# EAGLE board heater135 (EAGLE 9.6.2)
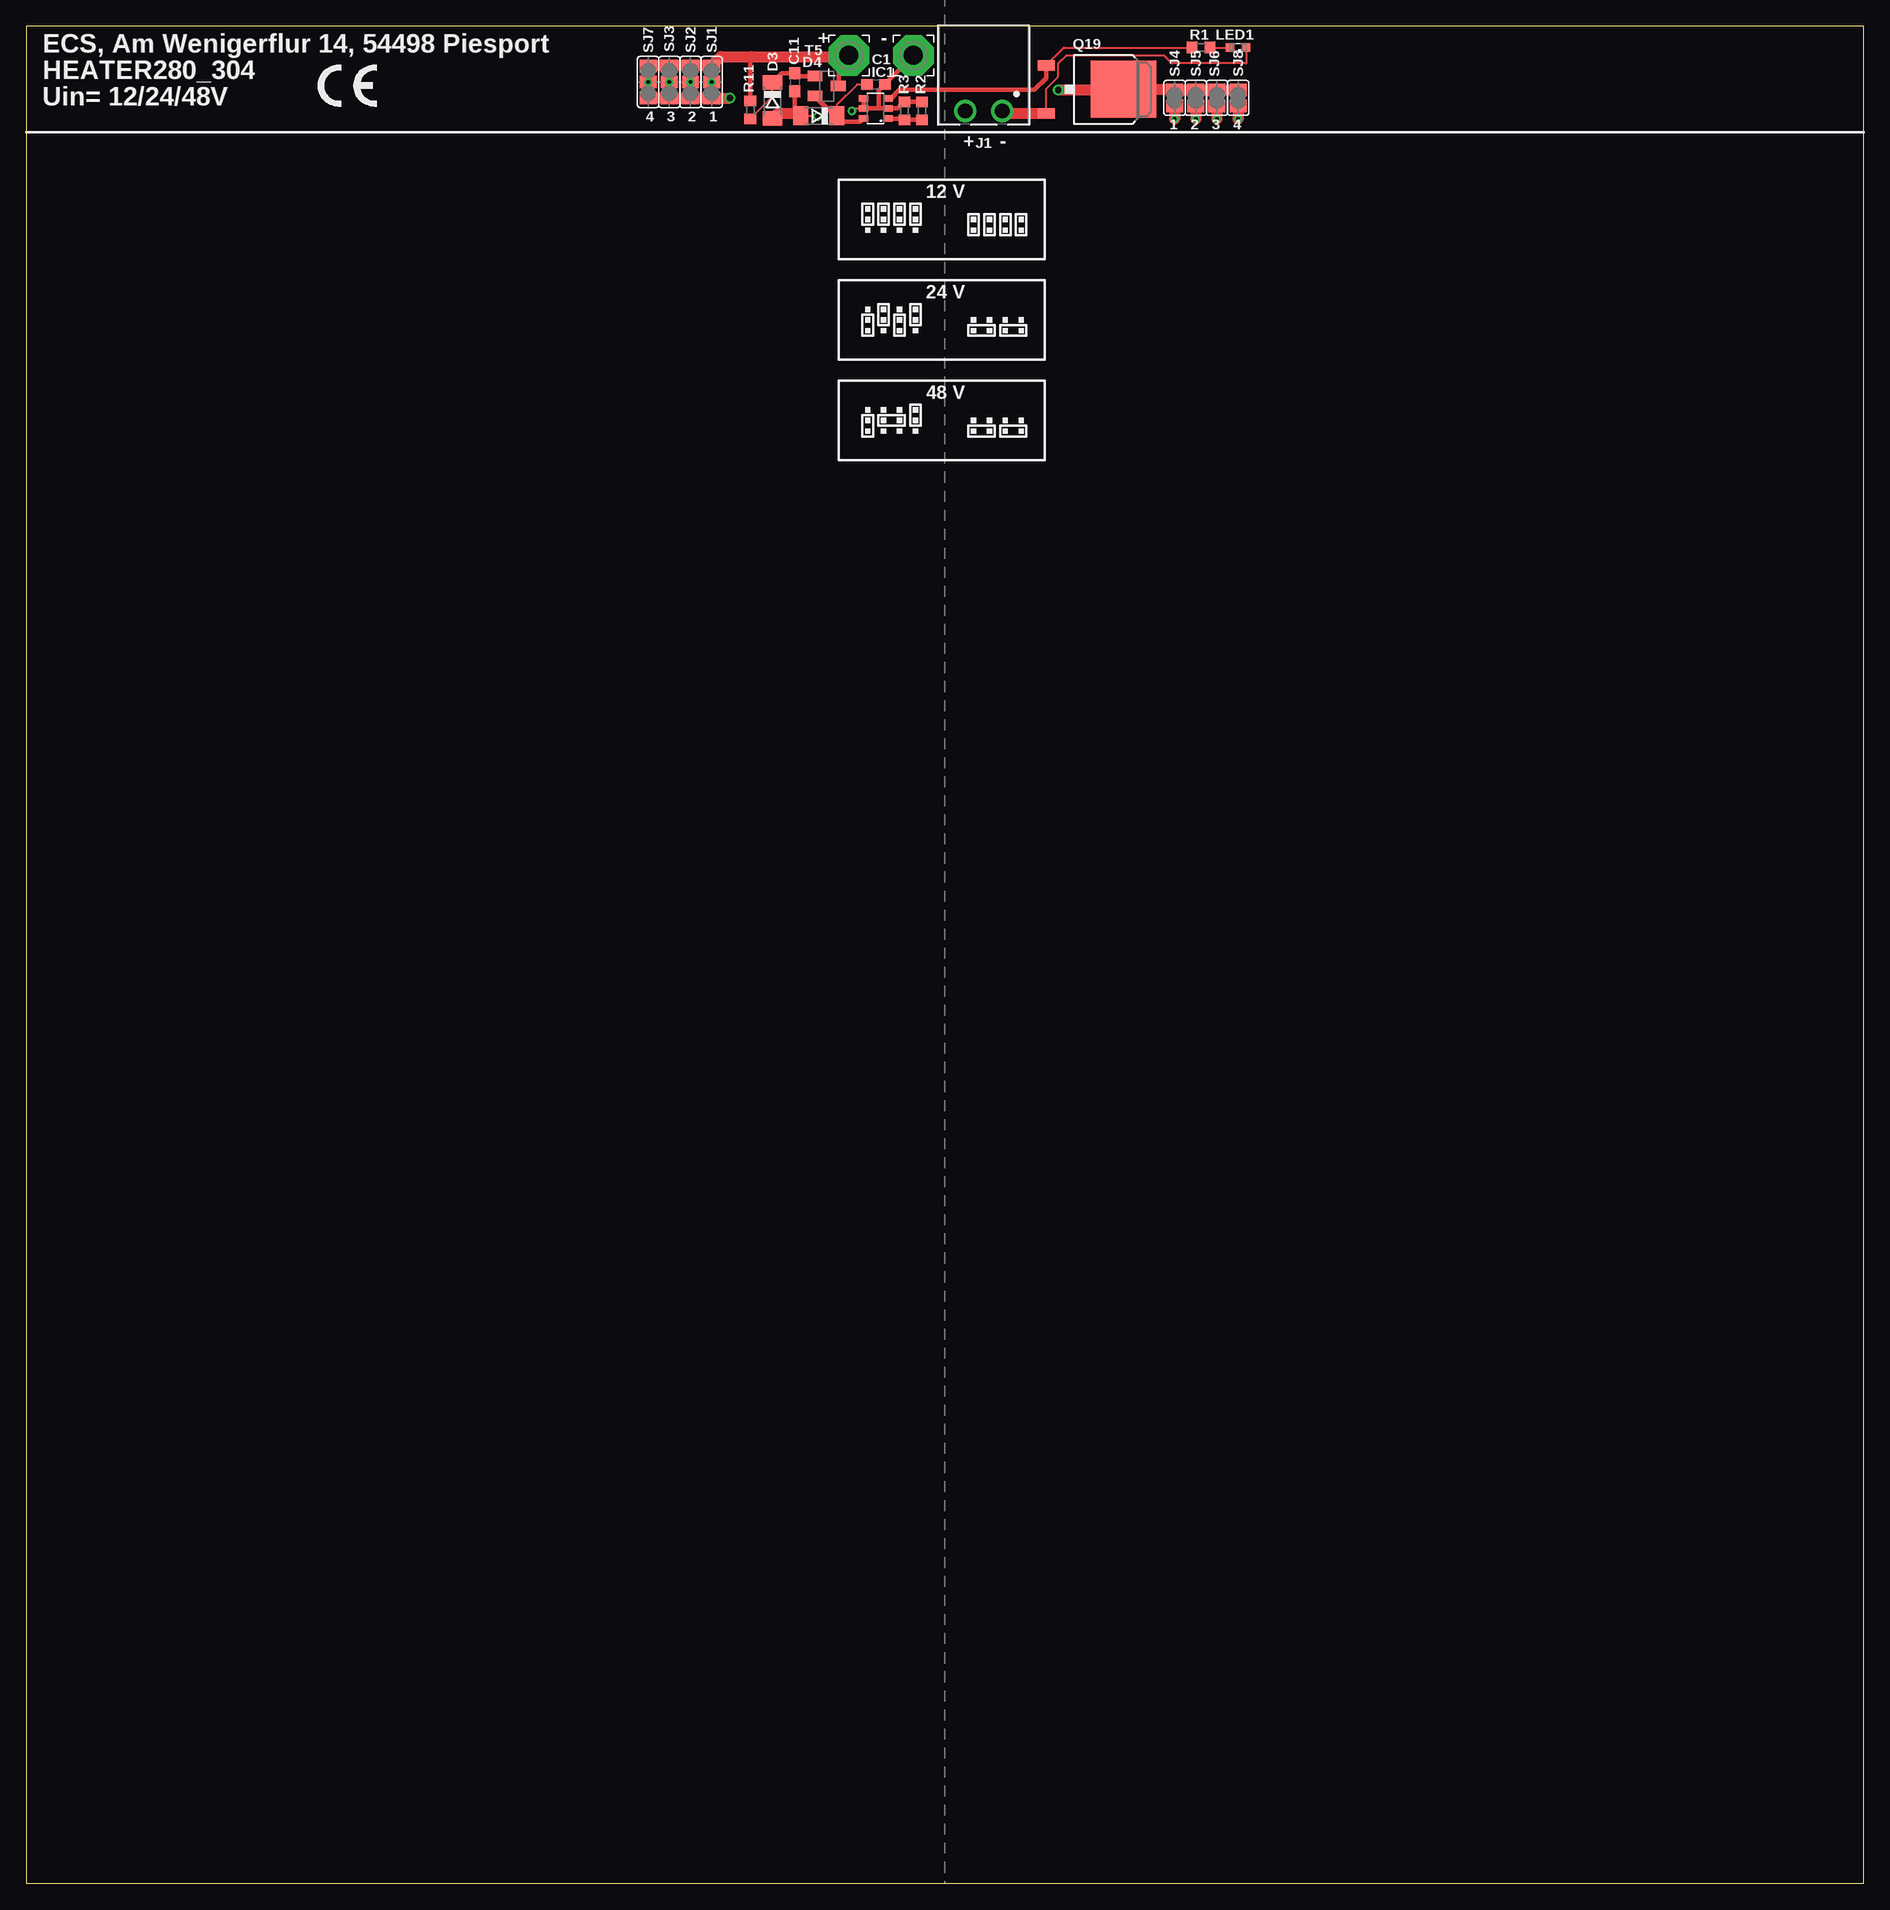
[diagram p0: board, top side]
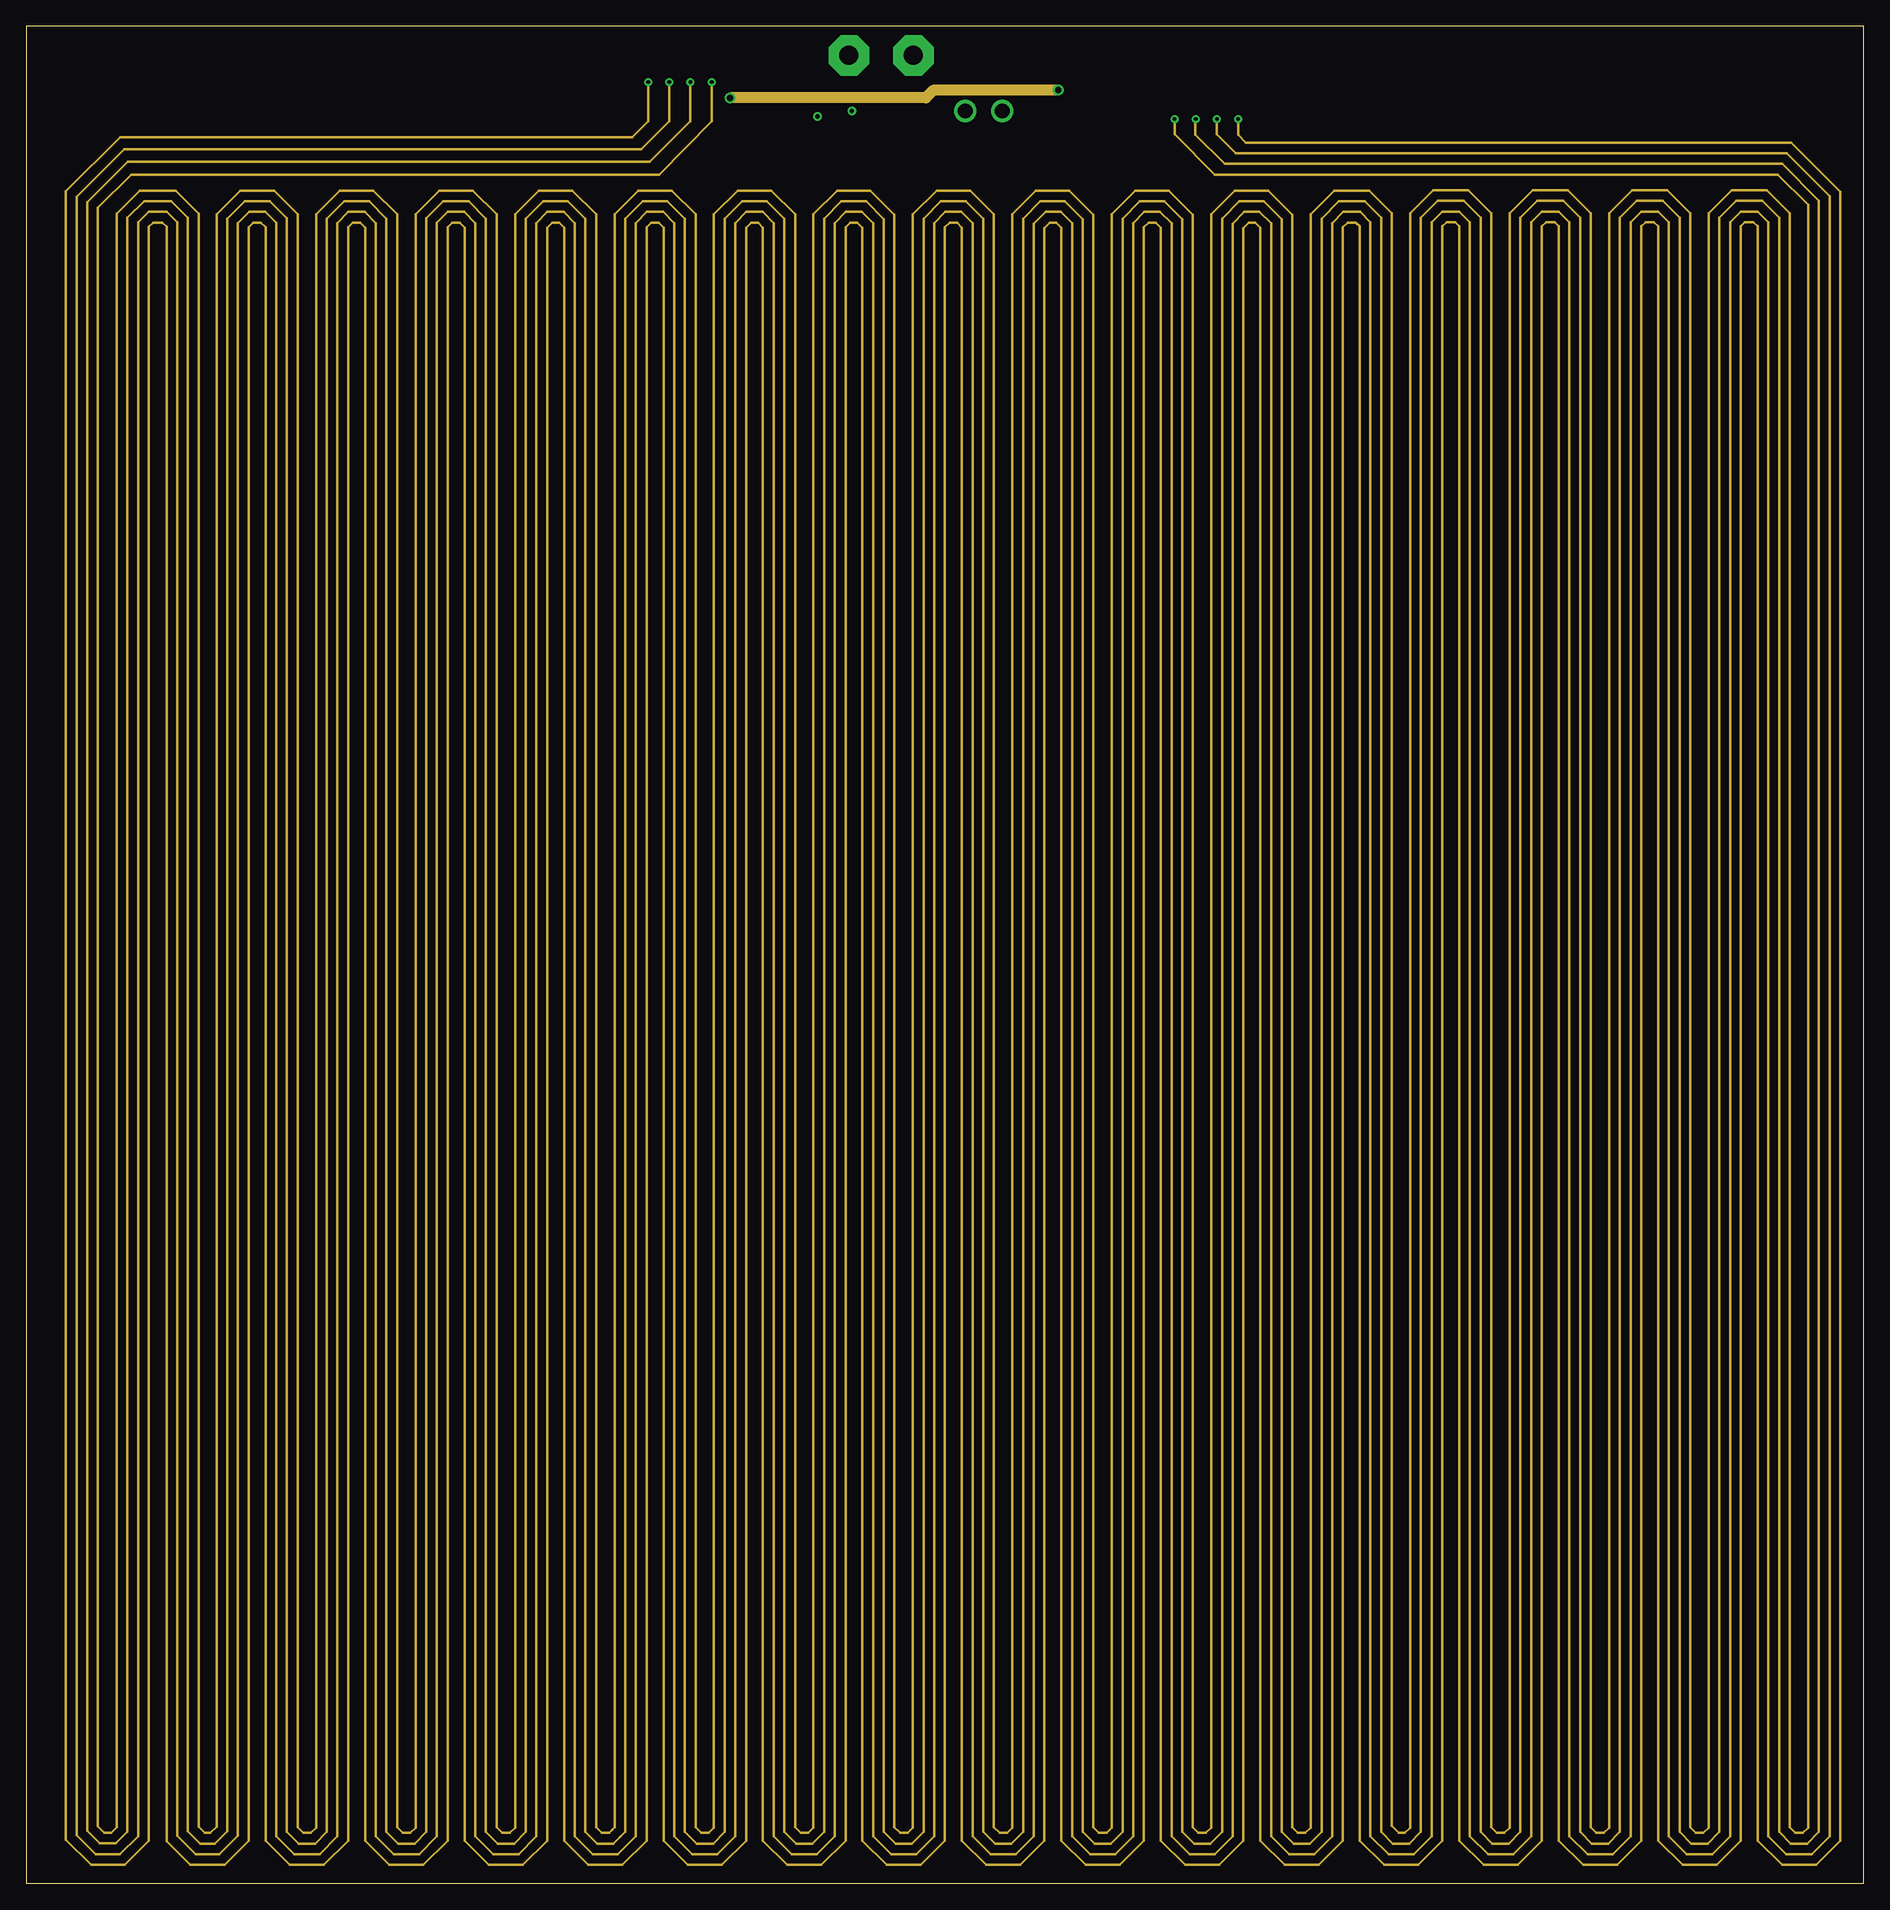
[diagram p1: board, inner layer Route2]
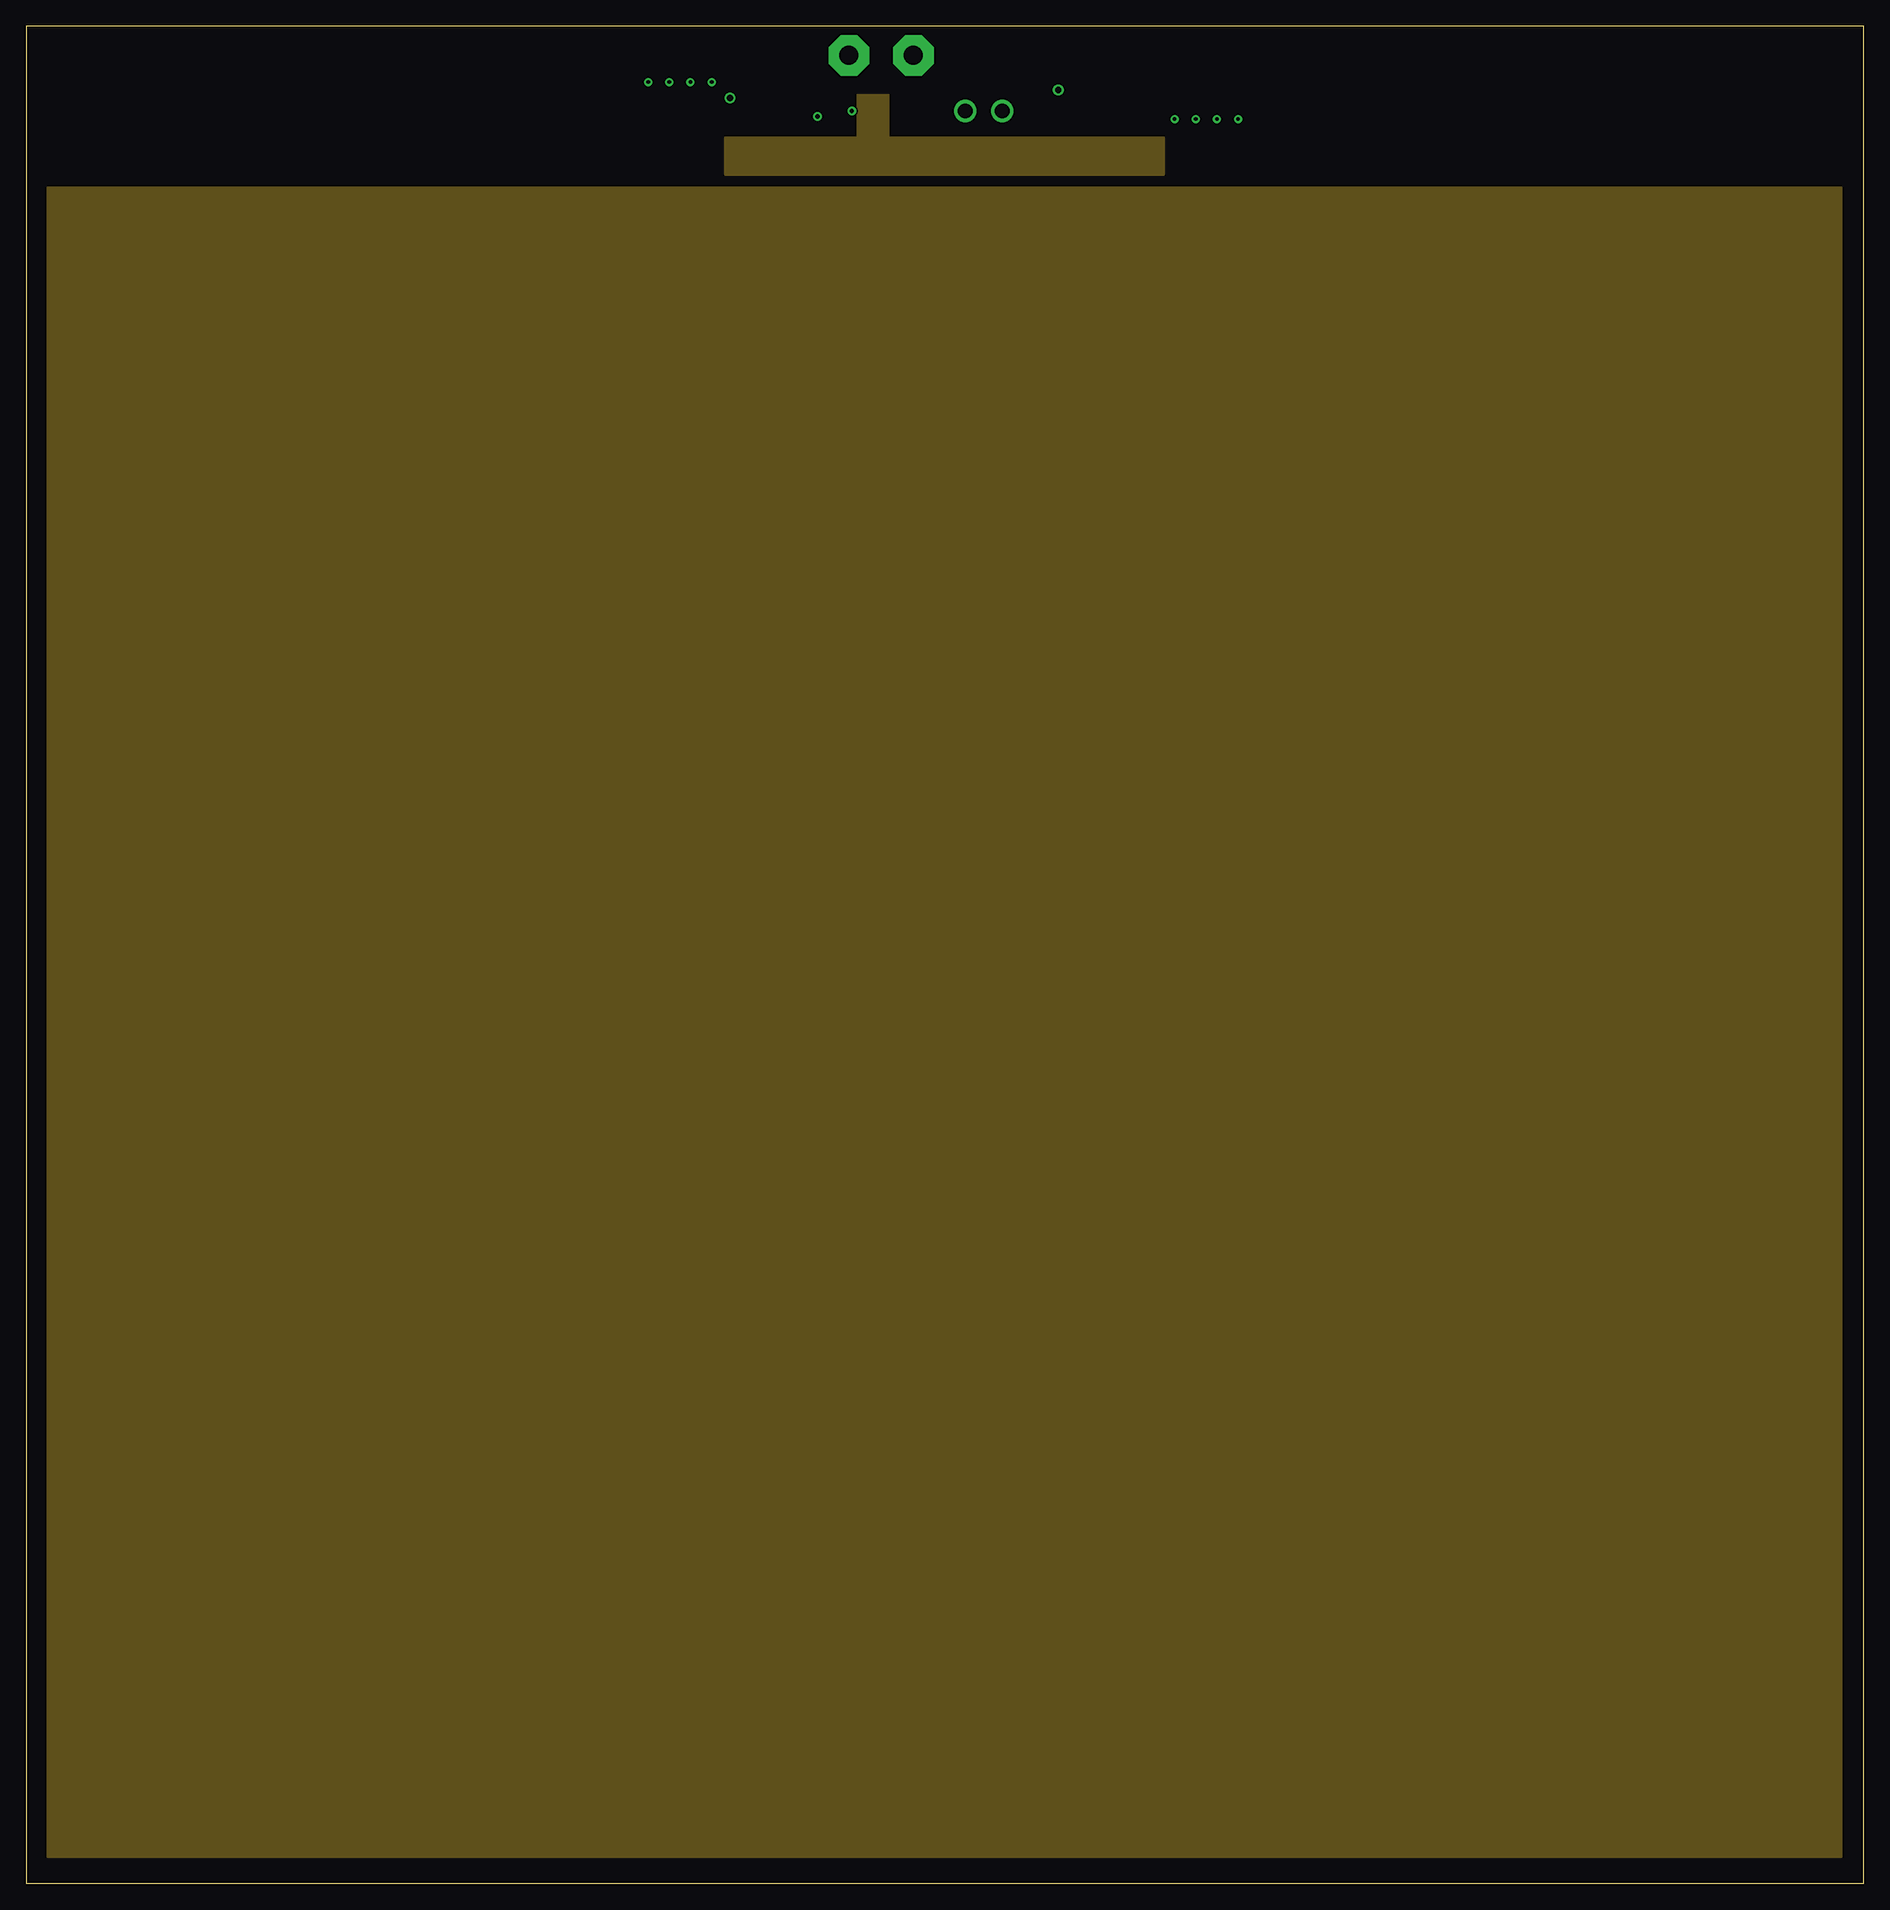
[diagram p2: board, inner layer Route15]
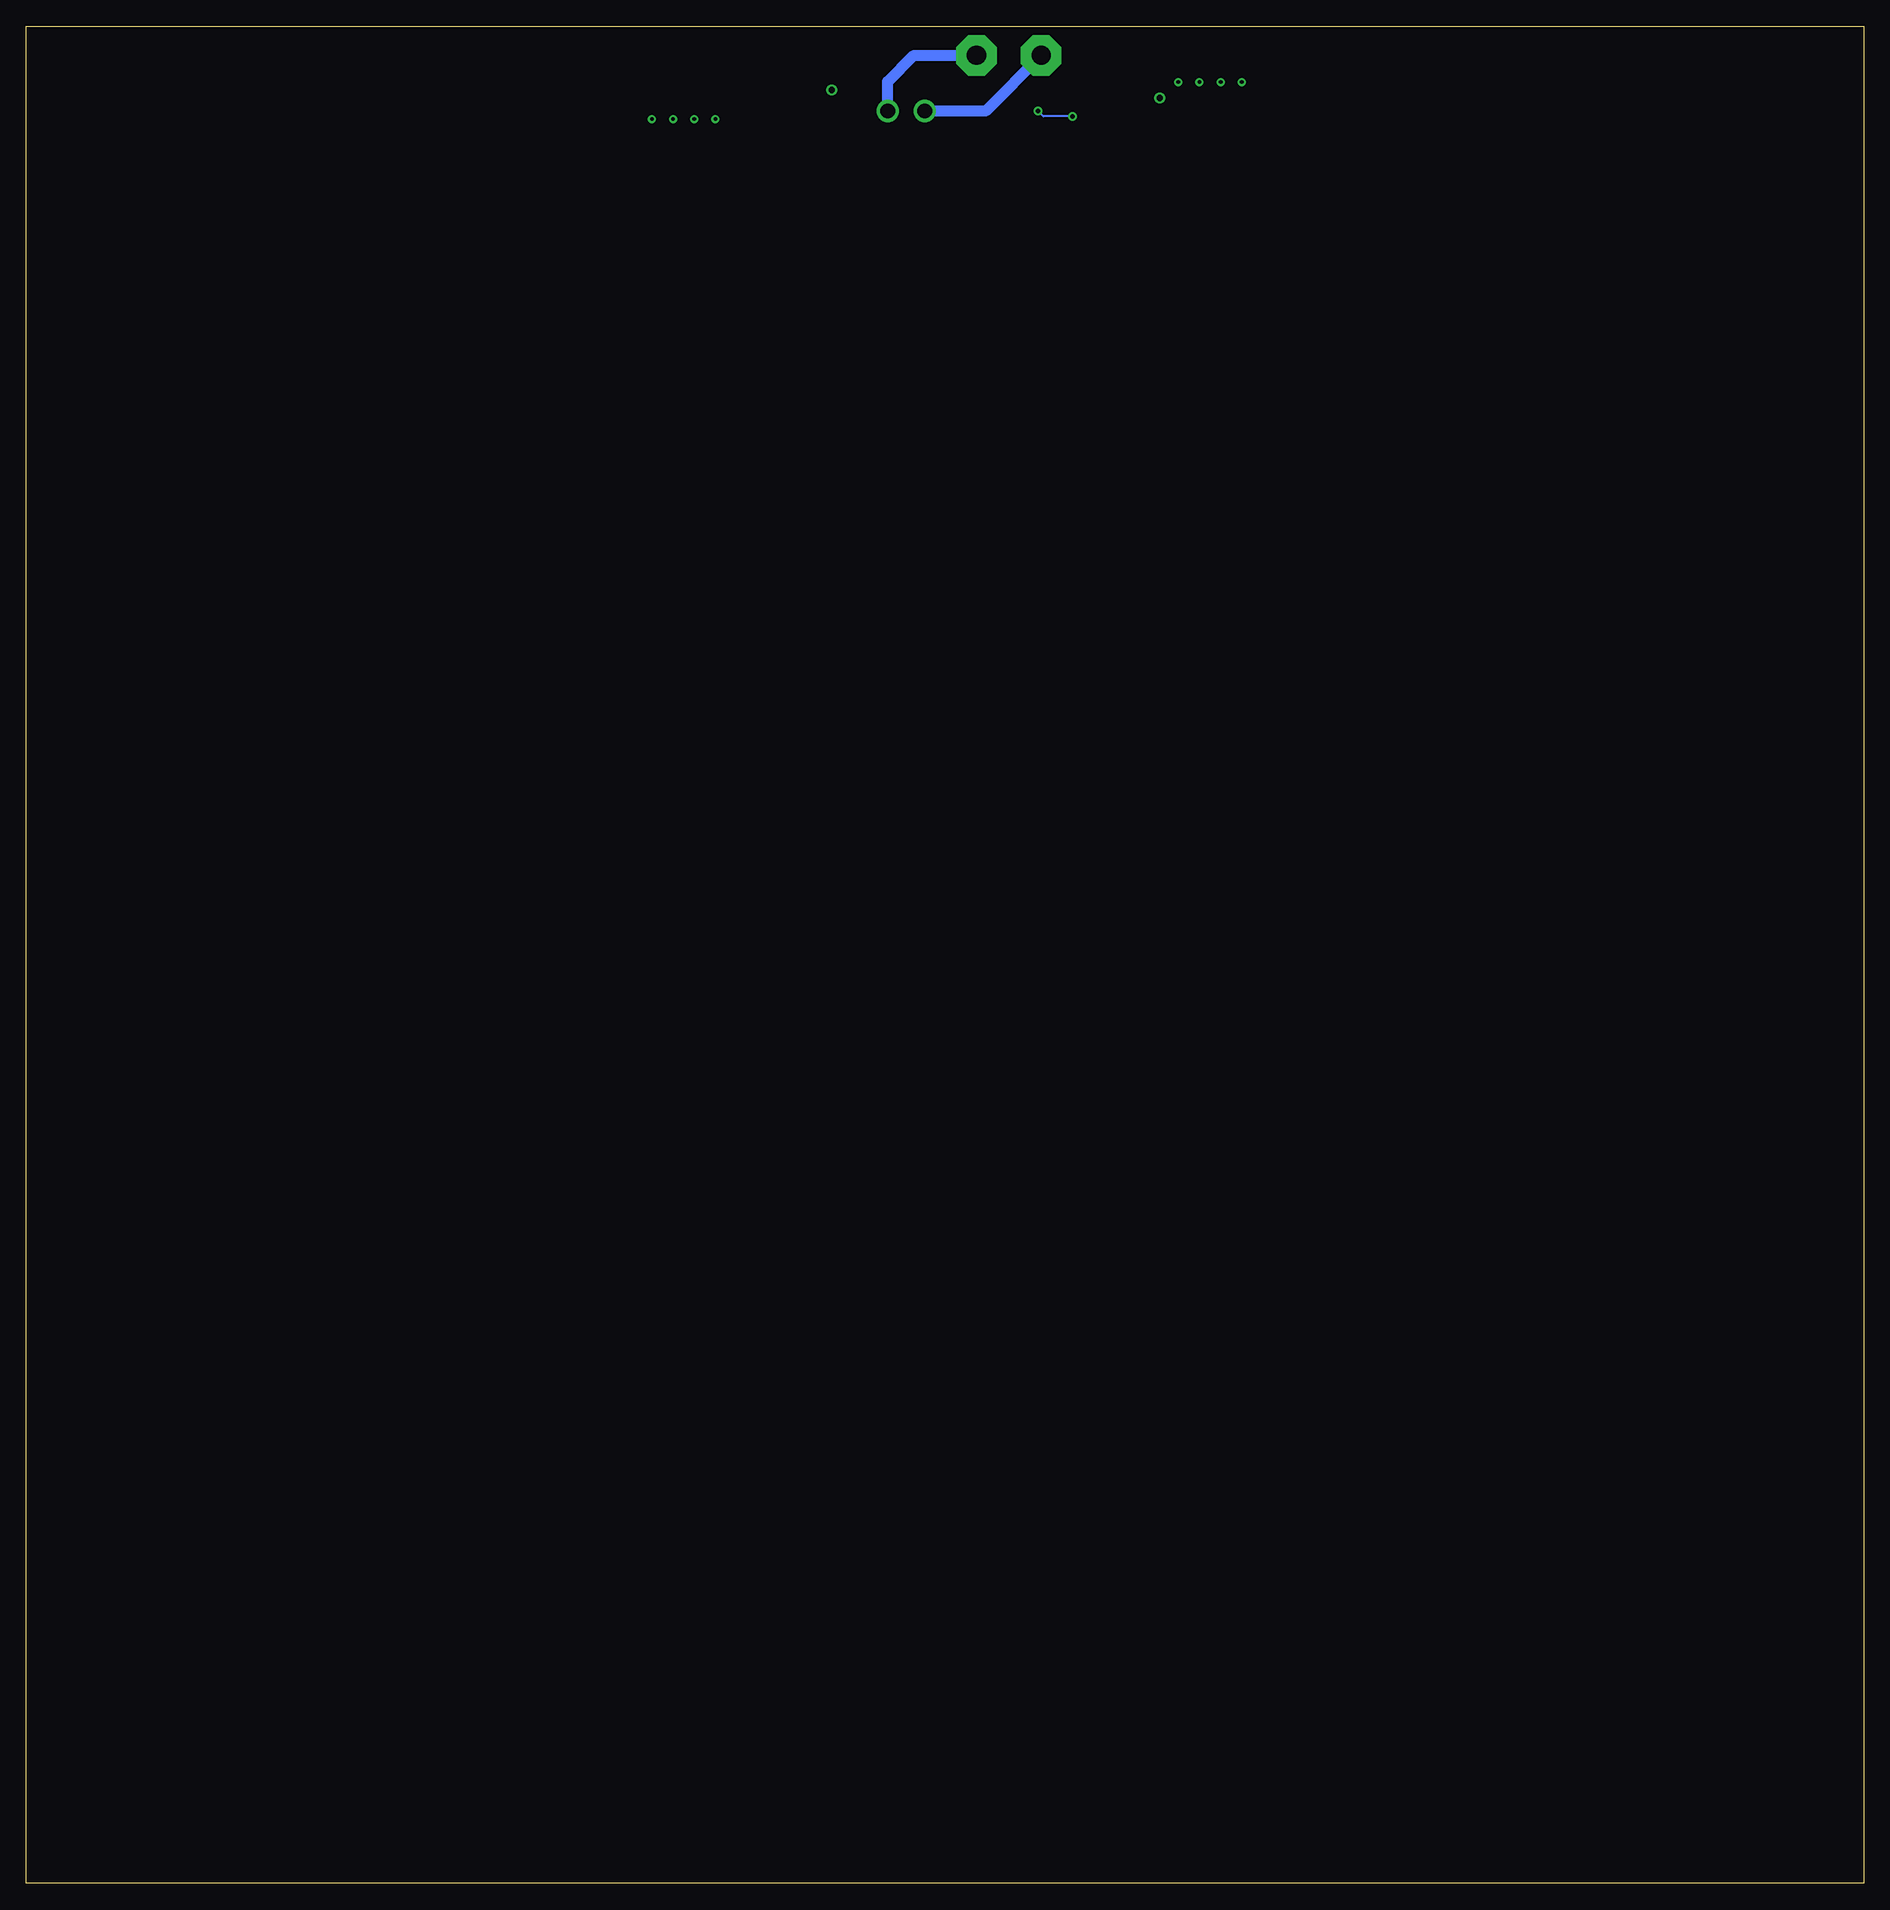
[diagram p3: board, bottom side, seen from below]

Size 173.6 x 175.5 mm. Coordinates in mm from the lower left corner, seen from the top.
Outline: 0,0 173.6,0 173.6,175.5 0,175.5 0,0
Copper layers (1+2*15+16): Top 0.035mm / dielectric 1.5mm / Route2 0.0175mm / dielectric 0.15mm / Route15 0.0175mm / dielectric 0.2mm / Bottom 0.035mm
Design rules "default *": minimum track width 6mil, minimum drill 0.35mm, track to track 6mil, track to pad 6mil, pad to pad 6mil, via to via 6mil, smd to smd 6mil, copper to edge 40mil, drill to drill 6mil, minimum pad ring 10mil, minimum via ring 8mil, stop-mask expansion 4mil, vias tented up to drill 0mil, thermal gap 10mil

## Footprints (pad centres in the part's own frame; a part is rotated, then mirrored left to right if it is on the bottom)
C0603 = smd 1.1 x 1: 1 -0.85,0; 2 0.85,0
SOD80C = smd 1.4 x 1.8: A 1.7,0; C -1.7,0
SOT23-6 = smd 0.6 x 0.9: 1 -0.95,-1.15; 2 0,-1.15; 3 0.95,-1.15; 4 0.95,1.15; 5 0,1.15; 6 -0.95,1.15
691322110002 = drill 1.4: 1 -1.75,0; 2 1.75,0
SML0603 = smd 0.8 x 0.8: A 0.75,0; C -0.75,0
3,81/1,4 = drill 1.8 pad 3.81 octagon: 1 0,0
D-PACK = smd 1 x 1.6: 1 -2.28,-4.8; 3 2.28,-4.8 | smd 5.4 x 6.2: 4 0,2.5
R0603 = smd 1 x 1.1: 1 -0.85,0; 2 0.85,0
SJ_2 = smd 1.168 x 1.6: 1 -1.524,0; 2 0,0; 3 1.524,0
SJ = smd 1.168 x 1.6: 1 -0.762,0; 2 0.762,0
SOT23-BEC = smd 1 x 1.4: B -0.95,-1.1; C 0,1.1; E 0.95,-1.1

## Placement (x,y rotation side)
C1  100n  [C0603]  80.27,170.02 0 top
C11  100n  [C0603]  72.6,170.23 270 top
D3  5V6  [SOD80C]  70.5,168.5 270 top
D4  5V1  [SOD80C]  74.88,167.05 180 top
IC1  MCP9510H  [SOT23-6]  80.25,167.75 90 top
J1  [691322110002]  90.46,167.51 180 top
LED1  [SML0603]  114.5,173.5 180 top
PAD1  [3,81/1,4]  77.72,172.76 0 top
PAD2  [3,81/1,4]  83.82,172.76 0 top
Q19  IRLR3110Z  [D-PACK]  101.16,169.55 270 top
R1  10k  [R0603]  111,173.5 180 top
R2  82k  [R0603]  84.64,167.52 270 top
R3  2M2  [R0603]  82.97,167.52 270 top
R11  100k  [R0603]  68.4,167.62 90 top
SJ1  [SJ_2]  64.75,170.25 90 top
SJ2  [SJ_2]  62.75,170.25 90 top
SJ3  [SJ_2]  60.75,170.25 90 top
SJ4  [SJ]  108.5,168.75 270 top
SJ5  [SJ]  110.5,168.75 270 top
SJ6  [SJ]  112.5,168.75 270 top
SJ7  [SJ_2]  58.75,170.25 90 top
SJ8  [SJ]  114.5,168.75 270 top
T5  BSR19A  [SOT23-BEC]  75.61,169.86 270 top
U$1  [CE-4MM]  27.5,167.88 0 top

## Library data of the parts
C1 C11 = rcl; PARTNO: C067; SPICEPREFIX: C
D3 = diode; PARTNO: D013
D4 = diode; PARTNO: D012
IC1 = mcp9509; PARTNO: IC333
J1 = Wurth_Connectors_WR-TBL Pluggable Connector; DATASHEET-URL: https://www.we-online.com/catalog/datasheet/691322110002.pdf; IR-UL: 10A; IR-VDE: 10.5A; MOUNT: THT; PART-NUMBER: 691322110002; PARTNO: CON212; PINS: 2; PITCH: 3.5mm; TYPE: Horizontal; WORKING-VOLTAGE-UL: 300V (AC); WORKING-VOLTAGE-VDE: 300V (AC)
LED1 = led; PARTNO: D078
PAD1 PAD2 = wirepad
Q19 = IRFR2607; PARTNO: T086
R1 = rcl; PARTNO: R221; SPICEPREFIX: R
R2 = rcl; PARTNO: R243; SPICEPREFIX: R
R3 = rcl; PARTNO: R277; SPICEPREFIX: R
R11 = rcl; PARTNO: R245; SPICEPREFIX: R
SJ1-SJ8 = jumper
T5 = transistor-neu-to92; PARTNO: T056
U$1 = logo

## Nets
+UB: J1.2 PAD1.1 R11.2 SJ1.3 SJ2.3 SJ3.3 SJ7.3 T5.C
GND: C1.2 C11.2 D3.A D4.A IC1.2 IC1.4 IC1.5 J1.1 LED1.C PAD2.1 Q19.3 R2.1 R3.1
N$1: IC1.3 Q19.1 R1.2
N$2: SJ1.2 SJ4.2
N$3: C11.1 D3.C R11.1 T5.B
N$4: IC1.1 R2.2 R3.2
N$5: C1.1 D4.C IC1.6 T5.E
N$6: LED1.A R1.1
N$7: SJ2.2 SJ5.2
N$8: SJ3.2 SJ6.2
N$9: SJ7.2 SJ8.2
N$11: Q19.4 SJ1.1 SJ2.1 SJ3.1 SJ4.1 SJ5.1 SJ6.1 SJ7.1 SJ8.1

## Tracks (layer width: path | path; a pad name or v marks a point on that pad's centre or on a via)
+UB
  Top 0.406: T5.C 76.75,169.9 76.75,171.79 77.61,172.65 PAD1.1 | R11.2 68.4,172.54 68.5,172.65
  Top 1.016: SJ7.3 SJ3.3 SJ2.3 SJ1.3 65.62,172.65 68.5,172.65 77.61,172.65
  Bottom 1.016: PAD1.1 82.97,167.51 J1.2
GND  (via drill 0.4)
  Top 0.2: LED1.C 115.25,172 108.25,172 107.5,172.75 98.25,172.75 97.5,172 97.5,170.75 96.36,169.61 Q19.3 | D4.A 74.7,167.05 v74.75,167 | v78,167.5 78.25,167.75 IC1.5
  Top 0.406: D4.A 72.6,167.63 C11.2 | 80.56,167.75 IC1.2 82.35,167.75 R3.1 R2.1 | 80.56,167.75 80.56,169.46 C1.2 81.12,170.06 PAD2.1 | IC1.4 IC1.5 80.56,167.75
  Top 1.016: D3.A 70.95,167.25 72.98,167.25 D4.A | Q19.3 92.45,167.27 J1.1
  Bottom 0.2: v74.75,167 77.5,167 v78,167.5
  Bottom 1.016: J1.1 92.21,170.29 89.74,172.76 PAD2.1
N$1
  Top 0.2: Q19.1 98.03,173.5 R1.2
  Top 0.406: IC1.3 81.7,168.7 82.5,169.5 95.25,169.5 96.36,170.61 Q19.1
N$2  (via drill 0.35, 0.35 pad 0.21)
  Top 1.016: SJ4.2 v108.5,166.75
  Route2 0.254: SJ1.2 64.75,166.52 59.79,161.5 9.9,161.5 6.75,158.35 6.75,5.37 7.37,4.76 8.01,4.76 8.54,5.28 8.54,157.82 10.71,159.99 14.09,159.99 16.26,157.82 16.26,5.32 16.84,4.75 17.38,4.75 17.97,5.34 17.97,157.76 20.2,159.99 23.41,159.99 25.63,157.77 25.63,5.27 26.16,4.75 26.86,4.75 27.37,5.25 27.37,157.76 29.6,159.99 32.79,159.99 35.03,157.75 35.03,5.27 35.55,4.75 36.26,4.75 36.77,5.25 36.77,157.77 38.99,159.99 42.19,159.99 44.43,157.75 44.43,5.27 44.95,4.75 45.66,4.75 46.17,5.25 46.17,157.76 48.4,159.99 51.59,159.99 53.83,157.75 53.83,5.27 54.35,4.75 55.05,4.75 55.35,5.05 55.57,5.27 55.57,157.76 57.8,159.99 60.99,159.99 63.23,157.75 63.23,5.27 63.75,4.75 64.47,4.75 64.97,5.25 64.97,157.76 67.2,159.99 70.39,159.99 72.63,157.75 72.63,5.27 73.16,4.75 73.86,4.75 74.37,5.25 74.37,157.76 76.6,159.99 79.75,159.99 82.03,157.72 82.03,5.27 82.56,4.75 83.26,4.75 83.77,5.25 83.77,157.76 86,159.99 89.19,159.99 91.43,157.75 91.43,5.27 91.95,4.75 92.66,4.75 93.17,5.25 93.17,157.76 95.4,159.99 98.56,159.99 100.83,157.72 100.83,5.27 101.35,4.75 102.07,4.75 102.57,5.25 102.57,157.76 104.8,159.99 107.95,159.99 110.23,157.72 110.23,5.27 110.75,4.75 111.46,4.75 111.97,5.25 111.97,157.76 114.2,159.99 117.36,159.99 119.63,157.72 119.63,5.27 120.16,4.75 120.86,4.75 121.37,5.25 121.37,157.76 123.6,159.99 126.89,159.99 129.03,157.85 129.03,5.42 129.7,4.75 130.26,4.75 130.77,5.25 130.77,157.85 132.94,160.03 136.25,160.03 138.43,157.85 138.43,5.27 138.96,4.75 139.66,4.75 140.17,5.25 140.17,157.85 142.34,160.03 145.66,160.03 147.83,157.85 147.83,5.27 148.35,4.75 149.06,4.75 149.57,5.25 149.57,157.85 151.75,160.03 155.06,160.03 157.23,157.85 157.23,5.27 157.75,4.75 158.46,4.75 158.97,5.25 158.97,157.85 161.15,160.03 164.46,160.03 166.63,157.85 166.63,5.27 167.16,4.75 167.86,4.75 168.37,5.25 168.37,158.63 165.5,161.5 112.3,161.5 108.5,165.3 v108.5,166.75
  other vias: 64.75,170.25
N$3
  Top 0.2: R11.1 70.5,168.87 D3.C
  Top 0.406: D3.C 71.38,171.08 C11.1 72.87,170.81 T5.B
N$4
  Top 0.406: IC1.1 82.97,166.8 R3.2 R2.2
N$5
  Top 0.2: C1.1 79.4,170 78.5,170 76.58,168.08 D4.C
  Top 0.406: T5.E 76.37,167.05 D4.C 76.83,166.8 76.95,166.8 77.25,166.5 78.77,166.5 IC1.6
N$6
  Top 0.2: R1.1 LED1.A
N$7  (via drill 0.35, 0.35 pad 0.21)
  Top 1.016: SJ5.2 v110.5,166.75
  Route2 0.254: SJ2.2 62.75,166.55 58.9,162.7 9.56,162.7 5.74,158.89 5.74,4.95 6.95,3.75 8.43,3.75 9.54,4.86 9.54,157.4 11.13,158.98 13.67,158.98 15.26,157.4 15.26,4.9 16.42,3.73 17.8,3.73 18.98,4.92 18.98,157.34 20.62,158.98 22.99,158.98 24.62,157.35 24.62,4.85 25.74,3.73 27.28,3.73 28.38,4.84 28.38,157.34 30.02,158.98 32.38,158.98 34.02,157.34 34.02,4.85 35.14,3.74 36.68,3.74 37.78,4.84 37.78,157.35 39.41,158.98 41.77,158.98 43.42,157.34 43.42,4.85 44.54,3.73 46.08,3.73 47.18,4.84 47.18,157.34 48.82,158.98 51.17,158.98 52.82,157.34 52.82,4.85 53.93,3.73 55.47,3.73 56.12,4.38 56.58,4.85 56.58,157.34 58.22,158.98 60.57,158.98 62.22,157.34 62.22,4.85 63.34,3.73 64.88,3.73 65.98,4.84 65.98,157.34 67.62,158.98 69.97,158.98 71.62,157.34 71.62,4.85 72.74,3.73 74.28,3.73 75.38,4.84 75.38,157.34 77.02,158.98 79.34,158.98 81.02,157.3 81.02,4.85 82.14,3.73 83.68,3.73 84.78,4.84 84.78,157.34 86.42,158.98 88.77,158.98 90.42,157.34 90.42,4.85 91.54,3.73 93.08,3.73 94.18,4.84 94.18,157.34 95.82,158.98 98.14,158.98 99.82,157.3 99.82,4.85 100.94,3.73 102.48,3.73 103.58,4.84 103.58,157.34 105.22,158.98 107.54,158.98 109.22,157.3 109.22,4.85 110.34,3.73 111.88,3.73 112.98,4.84 112.98,157.34 114.62,158.98 116.94,158.98 118.62,157.3 118.62,4.85 119.74,3.73 121.28,3.73 122.38,4.84 122.38,157.34 124.02,158.98 126.47,158.98 128.02,157.44 128.02,4.85 129.14,3.73 130.68,3.73 131.78,4.84 131.78,157.44 133.36,159.02 135.84,159.02 137.42,157.44 137.42,4.85 138.54,3.73 140.08,3.73 141.18,4.84 141.18,157.44 142.76,159.02 145.24,159.02 146.82,157.44 146.82,4.85 147.94,3.73 149.48,3.73 150.58,4.84 150.58,157.44 152.16,159.02 154.64,159.02 156.22,157.44 156.22,4.85 157.34,3.73 158.88,3.73 159.98,4.84 159.98,157.44 161.56,159.02 164.04,159.02 165.62,157.44 165.62,4.85 166.74,3.73 168.28,3.73 169.38,4.84 169.38,159.05 165.92,162.51 113.22,162.51 110.46,165.26 110.46,166.71
  Route2 0.4: 110.46,166.71 v110.5,166.75
  other vias: 62.75,170.25
N$8  (via drill 0.35, 0.35 pad 0.21)
  Top 1.016: SJ6.2 v112.5,166.75
  Route2 0.254: SJ3.2 60.75,166.55 58.1,163.9 9.23,163.9 4.74,159.41 4.74,4.53 6.54,2.73 8.84,2.73 10.55,4.45 10.55,156.98 11.54,157.97 13.26,157.97 14.24,156.98 14.24,4.48 16,2.73 18.22,2.73 19.99,4.5 19.99,156.93 21.04,157.97 22.57,157.97 23.61,156.94 23.61,4.43 25.32,2.73 27.7,2.73 29.39,4.42 29.39,156.93 30.43,157.97 31.96,157.97 33.01,156.92 33.01,4.43 34.72,2.73 37.1,2.73 38.79,4.42 38.79,156.94 39.83,157.97 41.36,157.97 42.41,156.92 42.41,4.43 44.12,2.73 46.5,2.73 48.19,4.42 48.19,156.93 49.24,157.97 50.76,157.97 51.81,156.92 51.81,4.43 53.52,2.73 55.88,2.73 57.59,4.43 57.59,156.93 58.64,157.97 60.16,157.97 61.21,156.92 61.21,4.43 62.92,2.73 65.3,2.73 66.99,4.42 66.99,156.93 68.04,157.97 69.56,157.97 70.61,156.92 70.61,4.43 72.32,2.73 74.7,2.73 76.39,4.42 76.39,156.93 77.44,157.97 78.92,157.97 80.01,156.88 80.01,4.43 81.72,2.73 84.1,2.73 85.79,4.42 85.79,156.93 86.84,157.97 88.36,157.97 89.41,156.92 89.41,4.43 91.12,2.73 93.5,2.73 95.19,4.42 95.19,156.86 96.3,157.97 97.72,157.97 98.81,156.88 98.81,4.43 100.52,2.73 102.9,2.73 104.59,4.42 104.59,156.93 105.64,157.97 107.12,157.97 108.21,156.88 108.21,4.43 109.92,2.73 112.3,2.73 113.99,4.42 113.99,156.86 115.1,157.97 116.52,157.97 117.61,156.88 117.61,4.43 119.32,2.73 121.7,2.73 123.39,4.42 123.39,156.93 124.44,157.97 126.06,157.97 127.01,157.02 127.01,4.43 128.72,2.73 131.1,2.73 132.79,4.42 132.79,157.02 133.78,158.01 135.42,158.01 136.41,157.02 136.41,4.43 138.12,2.73 140.5,2.73 142.19,4.42 142.19,157.02 143.18,158.01 144.82,158.01 145.81,157.02 145.81,4.43 147.52,2.73 149.9,2.73 151.59,4.42 151.59,157.02 152.58,158.01 154.22,158.01 155.21,157.02 155.21,4.43 156.92,2.73 159.3,2.73 160.99,4.42 160.99,157.02 161.98,158.01 163.62,158.01 164.61,157.02 164.61,4.43 166.32,2.73 168.7,2.73 170.39,4.42 170.39,159.47 166.34,163.52 114.28,163.52 112.5,165.3 v112.5,166.75
  other vias: 60.75,170.25
N$9  (via drill 0.35, 0.35 pad 0.21)
  Top 1.016: SJ8.2 v114.5,166.75
  Route2 0.254: SJ7.2 58.75,166.55 57.25,165.05 8.85,165.05 3.73,159.93 3.73,4.12 6.12,1.72 9.29,1.72 11.56,3.99 11.56,156.56 11.96,156.96 12.84,156.96 13.24,156.56 13.24,3.98 15.5,1.72 18.72,1.72 21,4 21,156.51 21.45,156.95 22.16,156.95 22.6,156.52 22.6,4.02 24.9,1.72 28.12,1.72 30.4,4 30.4,156.51 30.85,156.95 31.55,156.95 32,156.5 32,4.02 34.3,1.72 37.52,1.72 39.8,4 39.8,156.52 40.24,156.96 40.94,156.96 41.4,156.5 41.4,4.02 43.7,1.72 46.92,1.72 49.2,4 49.2,156.46 49.7,156.96 50.34,156.96 50.8,156.5 50.8,4 53.1,1.72 56.3,1.72 58.6,4 58.6,156.51 59.05,156.95 59.75,156.95 60.2,156.5 60.2,4.02 62.5,1.72 65.72,1.72 68,4 68,156.46 68.5,156.96 69.14,156.96 69.6,156.5 69.6,4.02 71.9,1.72 75.12,1.72 77.4,4 77.4,156.51 77.86,156.96 78.5,156.96 79,156.46 79,4.02 81.3,1.72 84.52,1.72 86.8,4 86.8,156.51 87.25,156.96 87.94,156.96 88.4,156.5 88.4,4.02 90.7,1.72 93.92,1.72 96.2,4 96.2,156.44 96.72,156.96 97.3,156.96 97.8,156.46 97.8,4.02 100.1,1.72 103.32,1.72 105.6,4 105.6,156.51 106.06,156.96 106.7,156.96 107.2,156.46 107.2,4.02 109.5,1.72 112.72,1.72 115,4 115,156.44 115.52,156.96 116.1,156.96 116.6,156.46 116.6,4.02 118.9,1.72 122.12,1.72 124.4,4 124.4,156.51 124.86,156.96 125.64,156.96 126,156.6 126,4.02 128.3,1.72 131.52,1.72 133.8,4 133.8,156.6 134.2,157 135,157 135.4,156.6 135.4,4.02 137.7,1.72 140.92,1.72 143.2,4 143.2,156.6 143.6,157 144.4,157 144.8,156.6 144.8,4.02 147.1,1.72 150.32,1.72 152.6,4 152.6,156.6 153,157 153.8,157 154.2,156.6 154.2,4.02 156.5,1.72 159.72,1.72 162,4 162,156.6 162.4,157 163.2,157 163.6,156.6 163.6,4.02 165.9,1.72 169.12,1.72 171.4,4 171.4,159.88 166.75,164.53 115.22,164.53 114.5,165.25 v114.5,166.75
  other vias: 58.75,170.25
N$10
  pour Route15: 78.5,169 78.5,165 66,165 66,161.5 107.5,161.5 107.5,165 81.5,165 81.5,169
N$11  (via drill 0.6)
  Top 1.016: SJ7.1 SJ3.1 SJ2.1 SJ1.1 66.48,168.73 v66.5,168.75 | SJ8.1 SJ6.1 SJ5.1 SJ4.1 104.65,169.51 103.66,170.5 Q19.4 103.61,169.5 v97.5,169.5
  Route2 1.016: v66.5,168.75 85,168.75 85.75,169.5 v97.5,169.5
N$12
  pour Route15: 171.5,160.25 2,160.25 2,2.5 171.5,2.5

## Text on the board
tPlace: + | - | ECS, Am Wenigerflur 14, 54498 Piesport | HEATER280_304 | Uin= 12/24/48V | 4 | 3 | 2 | 1 | 1 | 2 | 3 | 4 | + | - | 12 V | 24 V | 48 V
